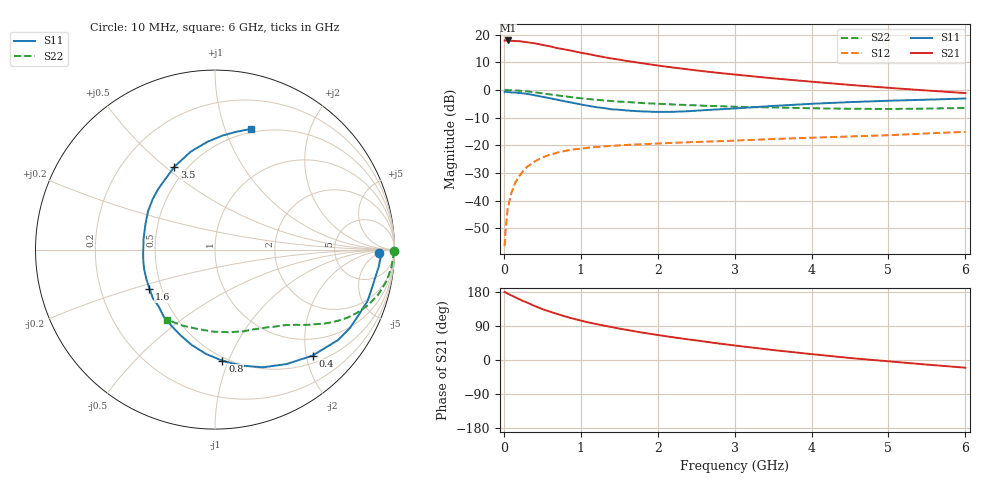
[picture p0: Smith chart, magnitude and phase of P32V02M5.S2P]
! SIEMENS Small Signal Semiconductors
! BFP181
! Si NPN RF Bipolar Junction Transistor in SOT143
! VCE = 2 V  IC = 2.5 mA
! Common Emitter S-Parameters:  March  1996
# GHz  S  MA  R  50
!  f  S11  S21  S12  S22
! GHz  MAG  ANG  MAG  ANG  MAG  ANG  MAG  ANG
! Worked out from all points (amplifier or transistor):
!   36 points, 10 MHz to 6 GHz, reference 50 ohm
!   highest |S21| = 17.9 dB at 50 MHz (marker M1)
!   |S21| within 3 dB of that: start of sweep to 742.1 MHz
!   unconditionally stable (mu >= 1): 2.188 GHz to end of sweep
!   at 250 MHz: K = 0.13, MSG = 23.4 dB, |S12| = -29.3 dB
!   at 1.4 GHz: K = 0.73, MSG = 15.8 dB, |S12| = -20.2 dB
!   at 6 GHz: K = 1.12, MAG = 4.9 dB, |S12| = -15.1 dB
!   S11 on the Smith chart (normalised r, x): 10 MHz: 21, -5; 400 MHz: 0.64, -2.12; 800 MHz: 0.47, -0.95; 1.6 GHz: 0.43, -0.23; 3.5 GHz: 0.43, +0.54; 6 GHz: 0.46, +1.23
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0.01  0.9141 -1.3  7.841 179.3  0.0015 79.9  0.9955 -0.5
0.02  0.924 -2.6  7.811 178.6  0.0026 82.2  0.9989 -1.2
0.05  0.9174 -5.9  7.846 175.1  0.0072 90.6  0.9921 -2.8
0.1  0.9018 -12.4  7.725 170.2  0.0141 82.7  0.9883 -5.5
0.2  0.8791 -24.6  7.618 160.4  0.0277 75.9  0.9694 -10.8
0.25  0.869 -30.4  7.441 155.7  0.0341 73.0  0.9546 -13.3
0.4  0.8027 -47.4  6.96 142.5  0.0509 63.0  0.9069 -20.0
0.5  0.7516 -58.1  6.532 134.4  0.06 57.5  0.8684 -23.8
0.6  0.7082 -67.8  6.142 127.5  0.0678 52.8  0.8308 -27.1
0.7  0.6626 -77.2  5.688 121.0  0.0739 48.9  0.7964 -29.7
0.8  0.6205 -86.2  5.376 114.9  0.0792 45.5  0.7651 -32.0
1  0.5476 -103.6  4.706 104.0  0.0869 39.8  0.7069 -35.9
1.1  0.5151 -111.8  4.453 99.1  0.0904 37.3  0.6847 -37.5
1.3  0.4703 -127.4  3.919 90.9  0.0955 33.8  0.6465 -40.4
1.6  0.4253 -149.1  3.339 79.4  0.1016 30.1  0.6056 -43.9
1.8  0.4098 -164.3  3.04 72.3  0.1043 28.4  0.5802 -46.3
2.2  0.4026 171.0  2.538 59.9  0.1106 25.4  0.5474 -51.4
2.8  0.4466 141.0  2.028 43.3  0.1186 22.7  0.5092 -59.7
3.5  0.5139 116.2  1.623 26.3  0.1296 20.2  0.482 -70.9
4.5  0.6027 93.9  1.233 5.3  0.1443 16.4  0.4572 -91.1
5.5  0.6672 79.7  0.977 -12.1  0.1636 13.5  0.4602 -112.9
6  0.7006 73.6  0.878 -20.3  0.1748 11.0  0.4727 -124.1
